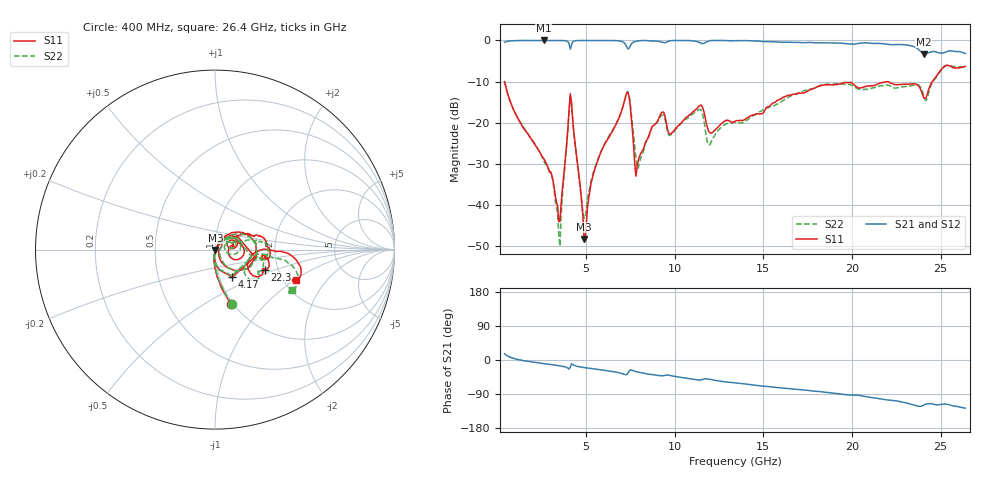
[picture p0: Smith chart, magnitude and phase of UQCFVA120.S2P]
!  Part Number  UQCFVA120  Mounting Orientation: Horizontal
!  Description: Ultra Low ESR Microwave capacitors
!  Application: Coupling, Bypass, Tuning, DC Block
!  Filters, Matching
# GHZ S DB R 50
! Freq  |S11|  S11 Ph  |S21|  S21 Ph  |S12|  S12 Ph  |S22|  S22 Ph
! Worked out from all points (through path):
!   401 points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, 400 MHz to 26.4 GHz, reference 50 ohm
!   highest |S21| = 0.00 dB at 2.61 GHz (marker M1); lowest = -3.3 dB at 24.06 GHz (marker M2)
!   group delay of S21, straight-line fit = 13.8 ps
!   lowest |S11| = -48.3 dB at 4.885 GHz (marker M3), VSWR 1.01, Z = 50.3 - j0.28 ohm
!   |S11| at or under -10 dB: start of sweep to 24.53 GHz
!   |S22| runs from -50.0 to -6.0 dB; largest |S21 - S12| = 0.0093
!   S11 on the Smith chart (normalised r, x): 400 MHz: 0.98, -0.66; 4.17 GHz: 1.15, -0.36; 22.3 GHz: 1.70, -0.41; 26.4 GHz: 2.35, -1.02
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0.4  -10.02 -73.4  -0.42 16.6  -0.42 16.5  -10.02 -73.0
2.61  -28.77 -97.2  0.00 -9.6  -0.01 -9.6  -29.27 -97.9
3.065  -32.83 -91.4  -0.01 -12.2  -0.01 -12.2  -32.73 -99.8
3.52  -44.04 1.0  -0.01 -15.4  0.00 -15.4  -50.04 4.3
3.975  -21.09 44.3  -0.30 -21.6  -0.31 -21.6  -21.54 44.3
4.17  -14.87 -57.6  -1.18 -10.0  -1.18 -10.6  -15.20 -57.0
4.755  -39.52 -87.0  -0.01 -18.9  -0.01 -19.1  -39.29 -74.0
4.885  -48.27 -46.2  -0.01 -19.9  -0.01 -20.0  -43.28 -29.3
5.535  -30.76 61.0  -0.01 -24.0  -0.01 -24.1  -30.46 47.9
7.29  -12.74 8.9  -1.51 -38.3  -1.49 -38.3  -12.75 7.0
7.875  -30.73 12.3  -0.17 -31.1  -0.17 -31.2  -31.13 -25.5
9.11  -18.89 42.8  -0.24 -41.1  -0.24 -41.2  -19.06 36.0
9.825  -22.55 23.9  -0.04 -41.7  -0.04 -41.7  -22.64 30.1
11.385  -15.93 2.9  -0.47 -52.9  -0.46 -53.0  -16.80 13.1
11.97  -22.40 -11.7  -0.08 -51.0  -0.09 -51.0  -25.42 14.6
13.4  -19.68 14.8  -0.04 -60.3  -0.05 -60.5  -19.93 19.9
17.755  -11.78 17.1  -0.52 -81.8  -0.54 -81.9  -11.72 9.8
22.11  -10.13 -20.4  -0.99 -106.0  -1.03 -106.1  -10.97 -24.7
22.305  -10.52 -21.9  -1.04 -106.7  -1.05 -106.8  -11.38 -26.8
24.06  -14.01 -25.3  -3.27 -118.7  -3.25 -118.8  -13.59 -38.5
25.23  -6.25 -11.5  -2.95 -116.1  -2.97 -116.2  -6.30 -17.2
26.4  -6.32 -20.2  -3.18 -127.1  -3.17 -127.2  -6.31 -28.1
